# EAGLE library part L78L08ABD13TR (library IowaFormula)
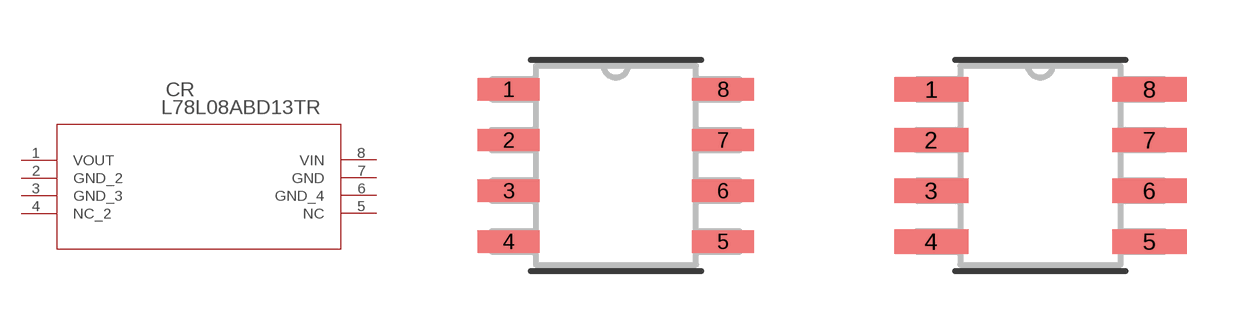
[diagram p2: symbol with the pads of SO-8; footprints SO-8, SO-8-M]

Designator prefix CR

## L78L08ABD13TR (MANUFACTURER_PART_NUMBER: L78L08ABD13TR; VENDOR: STMicroelectronics)  [SO-8]
1  VOUT  out
2  GND_2  pas
3  GND_3  pas
4  NC_2  nc
5  NC  nc
6  GND_4  pas
7  GND  pas
8  VIN  in

## L78L08ABD13TRSO-8-M (MANUFACTURER_PART_NUMBER: L78L08ABD13TR; VENDOR: STMicroelectronics)  [SO-8-M]
Pads as for SO-8

## L78L08ABD13TRSO-8-L (MANUFACTURER_PART_NUMBER: L78L08ABD13TR; VENDOR: STMicroelectronics)  [SO-8-L]
Pads as for SO-8

## Footprint SO-8 (pad centres in mm)
smd 1.549 x 0.559: 1 -2.68,1.905; 2 -2.68,0.635; 3 -2.68,-0.635; 4 -2.68,-1.905; 5 2.68,-1.905; 6 2.68,-0.635; 7 2.68,0.635; 8 2.68,1.905

## Footprint SO-8-M (pad centres in mm)
smd 1.854 x 0.61: 1 -2.731,1.905; 2 -2.731,0.635; 3 -2.731,-0.635; 4 -2.731,-1.905; 5 2.731,-1.905; 6 2.731,-0.635; 7 2.731,0.635; 8 2.731,1.905

## Footprint SO-8-L (pad centres in mm)
smd 1.245 x 0.508: 1 -2.629,1.905; 2 -2.629,0.635; 3 -2.629,-0.635; 4 -2.629,-1.905; 5 2.629,-1.905; 6 2.629,-0.635; 7 2.629,0.635; 8 2.629,1.905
